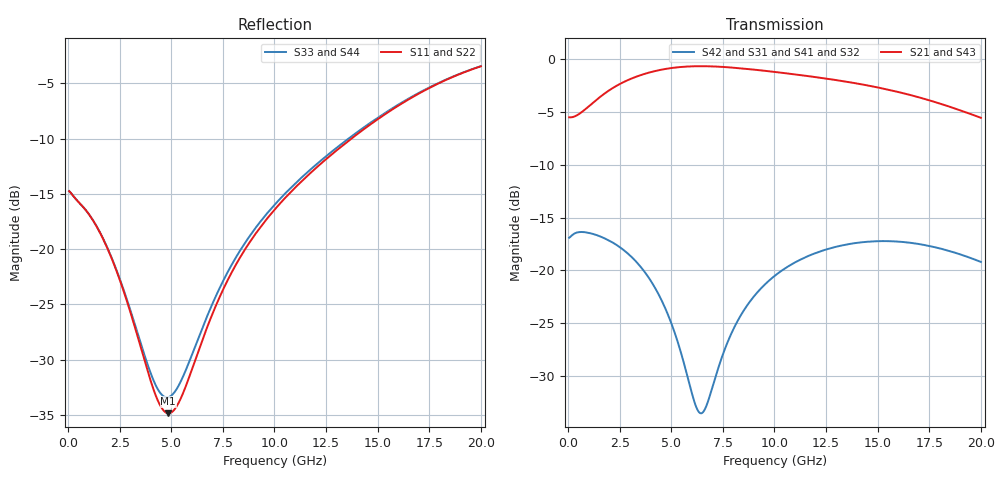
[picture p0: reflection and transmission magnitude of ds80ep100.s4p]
! Libra
! Texas Instruments S-Parameter Model for DS80EP100
! Model File Name: ds80ep100.s4p
! Date Created: 11/10/06
! Revision Number: 1.0
! Revision Notes:
! Created By: Koh, Yongseon
! Process Type: TYP
! Disclaimer:
! Copyright 2006 Texas Instruments Incorported. All rights reserved.
! This model is designed as an aid for customers of TEXAS INSTRUMENTS INCORPORATED ("TI") .
! TI and its licensors and suppliers make no warranties, either expressed
! or implied, with respect to this model, including the warranties of
! merchantability or fitness for a particular purpose.  The model is
! provided solely on an "as is" basis.  The entire risk as to its quality
! and performance is with the customer
! Notes Regarding Model:
! This model is a 4-port model in Libra or Touchstone format
! The differential input should be connected to port 1 and 3, and the
! differntial output should be connected to port 2 and 4.
# HZ  S  MA  R  50.0000
!freq (Hz)  mag("aaSP(1 1)")  phase("aaSP(1 1)") mag("aaSP(2 1)")  phase("aaSP(2 1)") mag("aaSP(3 1)")  phase("aaSP(3 1)") mag("aaSP(4 1)")  phase("aaSP(4 1)") mag("aaSP(1 2)")  phase("aaSP(1 2)") mag("aaSP(2 2)")  phase("aaSP(2 2)") mag("aaSP(3 2)")  phase("aaSP(3 2)") mag("aaSP(4 2)")  phase("aaSP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
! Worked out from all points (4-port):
!   400 points, 50 MHz to 20 GHz, reference 50 ohm
!   strongest paths, dB at 50 MHz, 5.05 GHz, 10.05 GHz, 15.05 GHz, 20 GHz:
!     S21: -5.5, -0.8, -1.2, -2.7, -5.5
!     S43: -5.5, -0.8, -1.2, -2.8, -5.6
!     S42: -16.9, -25.3, -20.5, -17.2, -19.2
!     S31: -16.9, -25.3, -20.5, -17.2, -19.2
!     S41: -16.9, -25.3, -20.4, -17.2, -19.2
!     S32: -16.9, -25.3, -20.4, -17.2, -19.2
!   lowest |S11| = -34.9 dB at 4.85 GHz (marker M1), VSWR 1.04, Z = 49 - j1.46 ohm
!   |S11| at or under -10 dB: start of sweep to 13.73 GHz
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5e7  0.1829 -2.9  0.5316 0.4  0.1428 0.0  0.1429 0.0
     0.5316 0.4  0.1829 -2.9  0.1429 0.0  0.1428 0.0
     0.1428 0.0  0.1429 0.0  0.1829 -2.9  0.5316 0.4
     0.1429 0.0  0.1428 0.0  0.5316 0.4  0.1829 -2.9
1.95e9  0.09863 -66.6  0.7093 4.7  0.1391 -35.4  0.1366 -34.6
        0.7093 4.7  0.09863 -66.6  0.1366 -34.6  0.1391 -35.4
        0.1391 -35.4  0.1366 -34.6  0.09908 -66.4  0.7098 4.7
        0.1366 -34.6  0.1391 -35.4  0.7098 4.7  0.09908 -66.4
4.85e9  0.01806 -124.4  0.9056 -19.9  0.06131 -83.2  0.06096 -82.3
        0.9056 -19.9  0.01806 -124.4  0.06096 -82.3  0.06131 -83.2
        0.06131 -83.2  0.06096 -82.3  0.02135 -119.5  0.9066 -20.1
        0.06096 -82.3  0.06131 -83.2  0.9066 -20.1  0.02135 -119.5
6.45e9  0.03748 -153.7  0.929 -34.9  0.02102 -44.4  0.02139 -43.3
        0.929 -34.9  0.03748 -153.7  0.02139 -43.3  0.02102 -44.4
        0.02102 -44.4  0.02139 -43.3  0.04262 -150.7  0.9284 -35.3
        0.02139 -43.3  0.02102 -44.4  0.9284 -35.3  0.04262 -150.7
8.45e9  0.09551 -182.4  0.9057 -52.3  0.06315 -10.4  0.06346 -10.4
        0.9057 -52.3  0.09551 -182.4  0.06346 -10.4  0.06315 -10.4
        0.06315 -10.4  0.06346 -10.4  0.1024 -181.5  0.9026 -52.7
        0.06346 -10.4  0.06315 -10.4  0.9026 -52.7  0.1024 -181.5
1.1e10  0.1897 -203.1  0.849 -72.3  0.1092 -41.1  0.1093 -41.1
        0.849 -72.3  0.1897 -203.1  0.1093 -41.1  0.1092 -41.1
        0.1092 -41.1  0.1093 -41.1  0.1978 -203.4  0.8429 -72.7
        0.1093 -41.1  0.1092 -41.1  0.8429 -72.7  0.1978 -203.4
2e10  0.672 -251.7  0.5288 -140.1  0.1097 -159.0  0.1097 -159.0
      0.5288 -140.1  0.672 -251.7  0.1097 -159.0  0.1097 -159.0
      0.1097 -159.0  0.1097 -159.0  0.6725 -252.2  0.523 -139.9
      0.1097 -159.0  0.1097 -159.0  0.523 -139.9  0.6725 -252.2
